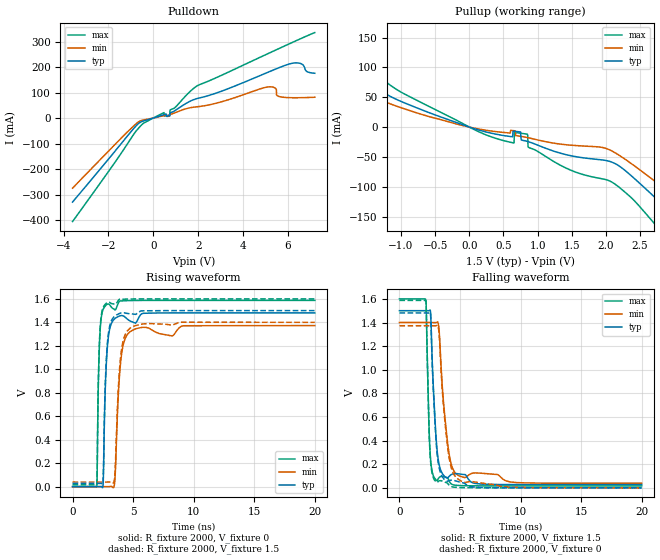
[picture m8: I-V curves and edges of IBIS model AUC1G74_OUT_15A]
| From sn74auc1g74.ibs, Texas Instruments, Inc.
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[Model]   AUC1G74_OUT_15A
Model_type  Output
Vref =   0
Rref =   2000
Cref =   15p
Vmeas =   0.75
| variable   typ   min   max
C_comp   5.00pF   0.17pF   14.09pF
| C_pullup   3.87pF   0.17pF   7.45pF
| C_pulldown   6.13pF   3.47pF   14.09pF
[Temperature Range]   40   100   -40
| Ambient temperature   25   85   -40
[Voltage range]   1.5   1.4   1.6
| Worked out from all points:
|   slope of the pulldown table from 0 to 0.225 V, typ, clamps not added: 37.2 ohm
|   slope of the pullup table from 0 to 0.225 V, typ, clamps not added: 29.5 ohm
|   rising waveform, R_fixture 2000, V_fixture 0: 20-80 % time 287ps typ, 424ps min, 190ps max; typ from 0 V to 1.48 V
|   falling waveform, R_fixture 2000, V_fixture 1.5: 20-80 % time 442ps typ, 678ps min, 253ps max; typ from 1.5 V to 0.027 V
|   rising waveform, R_fixture 2000, V_fixture 1.5: 20-80 % time 281ps typ, 413ps min, 188ps max; typ from 0.027 V to 1.5 V
|   falling waveform, R_fixture 2000, V_fixture 0: 20-80 % time 440ps typ, 682ps min, 251ps max; typ from 1.48 V to 0 V
[Pulldown]
| AUC1G74_OUT_15A
|   Voltage   I(typ)   I(min)   I(max)
-3.6V     -329.5mA   -274.8mA   -405.9mA
-570mV    -16.3mA    -10.82mA   -31.34mA
480mV     13.44mA    9.448mA    21.48mA
735mV     9.012mA    14.01mA    12.18mA
755mV     20.55mA    14.42mA    32.17mA
1.97V     76.83mA    44.37mA    127mA
5.095V    178.9mA    121.7mA    251.8mA
5.445V    191.6mA    116.7mA    266mA
5.495V    193.5mA    90.83mA    268.1mA
5.58V     196.5mA    85.25mA    271.5mA
6.39V     216.4mA    79.62mA    304mA
7.2V      175.6mA    81.55mA    335.1mA
[Pullup]
| AUC1G74_OUT_15A
|   Voltage   I(typ)   I(min)   I(max)
-3.6V     258.5mA    218.5mA    305.5mA
-3.035V   204.4mA    167.7mA    249.7mA
-2.21V    129.8mA    101.3mA    168.5mA
-935mV    39.88mA    29.96mA    54.57mA
395mV     -12mA      -7.71mA    -19.16mA
850mV     -24.02mA   -17.59mA   -11.85mA
870mV     -24.7mA    -18.1mA    -34.17mA
2.125V    -60.61mA   -42.44mA   -94.92mA
2.875V    -134.8mA   -104.7mA   -183.4mA
3.15V     -164.6mA   -129.3mA   -219.4mA
3.75V     -229.8mA   -184mA     -297mA
7.2V      -601mA     -503.3mA   -733.3mA
[Ramp]
| AUC1G74_OUT_15A
| variable   typ   min   max
dV/dt_r   0.89/2.93E-10   0.83/4.28E-10   0.95/1.93E-10
dV/dt_f   0.89/4.45E-10   0.82/6.82E-10   0.95/2.53E-10
R_load = 2000
[Rising Waveform]
| AUC1G74_OUT_15A
R_fixture =   2000
C_fixture =   0
L_fixture =   0
V_fixture =   0
V_fixture_min = 0
V_fixture_max = 0
|   Time   V(typ)   V(min)   V(max)
0s        8.172nV    30.93nV    915.6pV
2.005ns   -2.522uV   71.73nV    8.61mV
2.125ns   -8.737uV   -78.44nV   852.8mV
2.265ns   108.5uV    -263.1nV   1.31V
2.52ns    12.61mV    -5.014uV   1.509V
2.83ns    1.123V     -15.68uV   1.552V
3.45ns    1.428V     11.82mV    1.51V
3.98ns    1.457V     1.071V     1.583V
4.765ns   1.411V     1.322V     1.586V
20ns      1.481V     1.373V     1.587V
[Falling Waveform]
| AUC1G74_OUT_15A
R_fixture =   2000
C_fixture =   0
L_fixture =   0
V_fixture =   1.5
V_fixture_min = 1.4
V_fixture_max = 1.6
|   Time   V(typ)   V(min)   V(max)
0s        1.5V       1.4V       1.6V
2.195ns   1.5V       1.4V       1.588V
2.41ns    1.5V       1.4V       644mV
2.525ns   1.505V     1.4V       312.2mV
3.055ns   384.3mV    1.4V       63.73mV
3.26ns    205.5mV    1.353V     85.27mV
3.58ns    115.6mV    799.3mV    96.48mV
4.03ns    88.42mV    338.1mV    76.23mV
4.74ns    120.3mV    113.2mV    21.31mV
20ns      27.23mV    38.81mV    16.42mV
[Rising Waveform]
| AUC1G74_OUT_15A
R_fixture =   2000
C_fixture =   0
L_fixture =   0
V_fixture =   1.5
V_fixture_min = 1.4
V_fixture_max = 1.6
|   Time   V(typ)   V(min)   V(max)
0s        27.17mV    38.76mV    16.4mV
2.005ns   27.17mV    38.76mV    25.33mV
2.125ns   27.16mV    38.76mV    875.1mV
2.265ns   27.28mV    38.76mV    1.331V
2.52ns    43.03mV    38.76mV    1.525V
2.83ns    1.155V     38.75mV    1.567V
3.44ns    1.449V     51.18mV    1.555V
3.965ns   1.479V     1.102V     1.597V
4.745ns   1.473V     1.35V      1.599V
20ns      1.5V       1.4V       1.6V
[Falling Waveform]
| AUC1G74_OUT_15A
R_fixture =   2000
C_fixture =   0
L_fixture =   0
V_fixture =   0
V_fixture_min = 0
V_fixture_max = 0
|   Time   V(typ)   V(min)   V(max)
0s        1.481V     1.373V     1.587V
2.195ns   1.481V     1.373V     1.575V
2.415ns   1.48V      1.373V     606.9mV
2.525ns   1.486V     1.373V     293.2mV
3.06ns    349.8mV    1.373V     46.47mV
3.255ns   181.7mV    1.33V      57.81mV
3.58ns    87.76mV    769.2mV    56.18mV
4.035ns   58.22mV    299.2mV    30.78mV
4.83ns    53.37mV    74.54mV    3.549mV
20ns      58.88uV    35.25uV    23.83uV
